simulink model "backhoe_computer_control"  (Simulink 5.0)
settings: Solver=ode5  StartTime=0.0  StopTime=inf  FixedStep=0.001  RelTol=1e-3
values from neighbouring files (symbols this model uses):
  a1 = 8.5    [startup.m]
  a2 = 48    [startup.m]
  a3 = 38+11/16    (= 38.6875)    [startup.m]
  a4 = 18.5    [startup.m]
  Butter_Order = 2    [startup.m]
  c1 = [-0.0009634 -0.4050766 2.3355377]    [startup.m]
  c2 = [ -0.00644514 2.23812750 22.79925627]    [startup.m]
  c3 = [-0.0057802 2.2376391 22.8266324]    [startup.m]
  c4 = [-0.0020828 1.5286223 20.3434998]    [startup.m]
  R1A = 10    [startup.m]
  R1B = 35.875    [startup.m]
  R2C = 36    [startup.m]
  R2D = 9+7/8    (= 9.875)    [startup.m]
  R3F = 4.5    [startup.m]
  R3G = 5.5    [startup.m]
  REF = 29.625    [startup.m]
  RFH = 9.5    [startup.m]
  RGH = 9.5    [startup.m]
  T01A = acos(RAJ/R1A)    [startup.m]
  T12C = acos((a2^2 + R2C^2 - R1C^2)/(2*a2*R2C))    [startup.m]
  T23D = 0.1317    [startup.m]
  TB12 = acos((R1B^2 + a2^2 - R2B^2)/(2*a2*R1B))    [startup.m]
  TD23 = acos((R2D^2 + a3^2 - R3D^2)/(2*a3*R2D))    [startup.m]
  TDFE = 0.0503    [startup.m]
  TG34 = 1.6966    [startup.m]
undefined symbols (not defined in the file or in its folder): channels, ended, Single
libraries: dsparch4 x18, xpclib x5, simulink x5

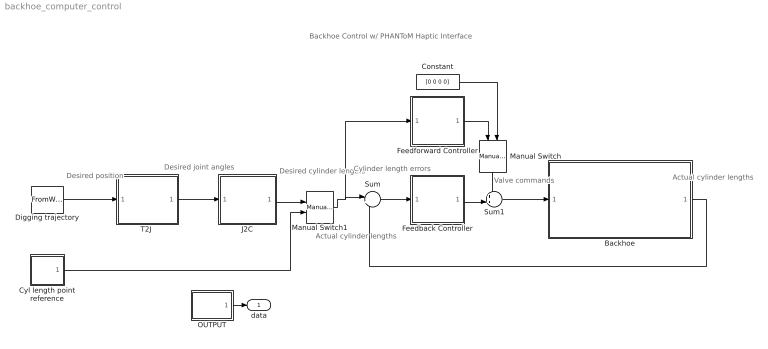
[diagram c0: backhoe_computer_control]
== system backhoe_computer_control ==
  note: Desired cylinder lengths
  note: Cylinder length errors
  note: Actual cylinder lengths
  note: Actual cylinder lengths
  note: Desired joint angles
  note: Desired position
  note: Backhoe Control w/ PHANToM Haptic Interface
  note: Valve commands
  Backhoe : Subsystem
  Constant : Constant  Value=[0 0 0 0]
  Cyl length point reference : Subsystem
  Digging trajectory : FromWorkspace  VariableName=traj  SampleTime=0  OutputAfterFinalValue=Holding final value
  Feedback Controller : Subsystem
  Feedforward Controller : Subsystem
  J2C : Subsystem
  Manual Switch : simulink/Signal Routing/Manual Switch  Orientation=down  sw=0  action=0
  Manual Switch1 : simulink/Signal Routing/Manual Switch  sw=0  action=0
  OUTPUT : Subsystem
  Sum : Sum  Inputs=|+-
  Sum1 : Sum  Inputs=++|
  "T2J " : Subsystem
  data : Outport
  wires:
  Sum/1 -> Feedback Controller/1(e)
  Backhoe/1(yc) -> Sum/2
  "T2J "/1(qdes) -> J2C/1(qdes)
  Feedback Controller/1(Us) -> Sum1/2
  Sum1/1 -> Backhoe/1(Us)
  Manual Switch/1 -> Sum1/1
  Feedforward Controller/1(UsFF) -> Manual Switch/1
  Constant/1 -> Manual Switch/2
  Digging trajectory/1 -> "T2J "/1(yp)
  J2C/1(ycdes) -> Manual Switch1/1
  Manual Switch1/1 -> Sum/1, Feedforward Controller/1(ycdes)
  Cyl length point reference/1(ycdes) -> Manual Switch1/2
  OUTPUT/1(datalog) -> data/1

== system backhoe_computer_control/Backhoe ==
  note: Valve commands
  note: Position sensor signals
  note: Cylinder lengths
  Us : Inport
  Anti-Deadband Block : Subsystem
  Backhoe Interface : Subsystem
  Position sensor conversions : Subsystem
  "Vpres -> p  conversion" : Lookup  InputValues=[2 10]  OutputValues=[0 3000]  ShowAdditionalParam=on  LookUpMeth=Interpolation-Use End Values
  yc : Outport
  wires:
  Backhoe Interface/1(Vpos) -> Position sensor conversions/1(Vc)
  Position sensor conversions/1(yc) -> yc/1, [GLOBAL_yc]
  Us/1 -> Anti-Deadband Block/1(us)
  Backhoe Interface/2(Vpres) -> "Vpres -> p  conversion"/1
  Anti-Deadband Block/1(Us) -> Backhoe Interface/1(Us)
  "Vpres -> p  conversion"/1 -> [GLOBAL_p]

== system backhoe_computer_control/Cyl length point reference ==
  Boom : Sin  Amplitude=0  Bias=31  Frequency=2*pi*0.1  SampleTime=0
  Bucket : Sin  Amplitude=0  Bias=32  Frequency=2*pi*0.1  SampleTime=0
  Mux2 : Mux
  Stick : Sin  Amplitude=0  Bias=33  Frequency=2*pi*0.1  SampleTime=0
  Swing : Sin  Amplitude=0  Frequency=2*pi*0.1  SampleTime=0
  ycdes : Outport
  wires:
  Swing/1 -> Mux2/1
  Bucket/1 -> Mux2/4
  Stick/1 -> Mux2/3
  Boom/1 -> Mux2/2
  Mux2/1 -> ycdes/1

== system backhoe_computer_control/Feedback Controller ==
  e : Inport
  Demux : Demux
  Mux : Mux
  "boom [in/s] -> [V]" : Lookup  InputValues=[-1 0 1]  OutputValues=[-0.05 0 0.6]  ShowAdditionalParam=on
  "bucket [in/s] -> [V]" : Lookup  InputValues=[-1 0 1]  OutputValues=[-0.2 0 0.2]  ShowAdditionalParam=on
  "stick [in/s] -> [V]" : Lookup  InputValues=[-1 0 1]  OutputValues=[-0.2 0 0.2]  ShowAdditionalParam=on
  "swing [rad/s] -> [V]" : Lookup  InputValues=[-1 0 1]  OutputValues=[-0.2 0 0.2]  ShowAdditionalParam=on
  Us : Outport
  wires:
  e/1 -> Demux/1
  Demux/1 -> "swing [rad/s] -> [V]"/1
  "swing [rad/s] -> [V]"/1 -> Mux/1
  Demux/2 -> "boom [in/s] -> [V]"/1
  "boom [in/s] -> [V]"/1 -> Mux/2
  Demux/3 -> "stick [in/s] -> [V]"/1
  "stick [in/s] -> [V]"/1 -> Mux/3
  Demux/4 -> "bucket [in/s] -> [V]"/1
  "bucket [in/s] -> [V]"/1 -> Mux/4
  Mux/1 -> Us/1

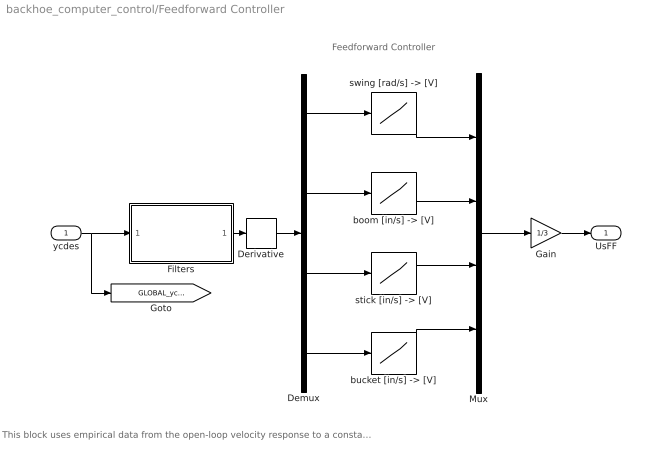
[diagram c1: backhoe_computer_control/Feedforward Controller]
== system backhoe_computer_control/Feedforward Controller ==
  note: This block uses empirical data from the open-loop velocity response to a constant voltage command to the valves. Relationships have been inverted to determine the required voltage to produce a desired velocity for each function.
  note: Feedforward Controller
  ycdes : Inport
  Demux : Demux
  Derivative : Derivative
  Filters : Subsystem
  Gain : Gain  Gain=1/3
  Mux : Mux
  "boom [in/s] -> [V]" : Lookup  InputValues=[-1.0 0 3.0]  OutputValues=[-0.25 0 0.25]  ShowAdditionalParam=on
  "bucket [in/s] -> [V]" : Lookup  InputValues=[-2.3 0 2.75]  OutputValues=[-0.25 0 0.25]  ShowAdditionalParam=on
  "stick [in/s] -> [V]" : Lookup  InputValues=[-1.6 0 1.75]  OutputValues=[-0.25 0 0.25]  ShowAdditionalParam=on
  "swing [rad/s] -> [V]" : Lookup  InputValues=[-0.6 0 0.7]  OutputValues=[-0.25 0 0.25]  ShowAdditionalParam=on
  UsFF : Outport
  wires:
  ycdes/1 -> Filters/1(unfiltered), [GLOBAL_ycdes]
  Derivative/1 -> Demux/1
  Demux/1 -> "swing [rad/s] -> [V]"/1
  "swing [rad/s] -> [V]"/1 -> Mux/1
  Demux/2 -> "boom [in/s] -> [V]"/1
  "boom [in/s] -> [V]"/1 -> Mux/2
  Demux/3 -> "stick [in/s] -> [V]"/1
  "stick [in/s] -> [V]"/1 -> Mux/3
  Demux/4 -> "bucket [in/s] -> [V]"/1
  "bucket [in/s] -> [V]"/1 -> Mux/4
  Mux/1 -> Gain/1
  Filters/1(filtered) -> Derivative/1
  Gain/1 -> UsFF/1

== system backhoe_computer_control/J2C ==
  note: Joint Space -> Cylinder Space Transformation
  note: Swing Cylinders
  qdes : Inport
  Boom cylinder : Subsystem
  Bucket cylinder : Subsystem
  Demux : Demux
  Mux : Mux
  Stick cylinder : Subsystem
  overswing  protection : Saturate  UpperLimit=pi/3  LowerLimit=-pi/2
  ycdes : Outport
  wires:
  qdes/1 -> Demux/1
  Mux/1 -> ycdes/1
  Demux/2 -> Boom cylinder/1(q2)
  Boom cylinder/1(yc3) -> Mux/2
  Demux/3 -> Stick cylinder/1(q3)
  Stick cylinder/1(yc4) -> Mux/3
  Demux/4 -> Bucket cylinder/1(q4)
  Bucket cylinder/1(yc5) -> Mux/4
  Demux/1 -> overswing  protection/1
  overswing  protection/1 -> Mux/1

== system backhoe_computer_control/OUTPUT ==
  Clock : Clock
  Mux : Mux  Inputs=5
  "Scope (xPC) " : xpclib/Misc./Scope (xPC)   scopeno=2  scopetype=Target  viewmode=Graphical redraw  grid=on  ylimits=[0,0]  autostart=on  nosamples=500  noprepostsamples=0  interleave=1  triggermode=FreeRun  triggersignal=1  triggerlevel=0.0  triggerslope=either  triggerscope=1  triggersample=0
  Scope (xPC) 1 : xpclib/Misc./Scope (xPC)   scopeno=3  scopetype=Target  viewmode=Graphical redraw  grid=on  ylimits=[0,0]  autostart=on  nosamples=500  noprepostsamples=0  interleave=1  triggermode=FreeRun  triggersignal=1  triggerlevel=0.0  triggerslope=either  triggerscope=1  triggersample=0
  Scope (xPC) 2 : xpclib/Misc./Scope (xPC)   scopeno=1  scopetype=Target  viewmode=Graphical redraw  grid=on  ylimits=[0,0]  autostart=on  nosamples=500  noprepostsamples=0  interleave=1  triggermode=FreeRun  triggersignal=1  triggerlevel=0.0  triggerslope=either  triggerscope=1  triggersample=0
  Selector : Selector  InputPortWidth=4
  datalog : Outport
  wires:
  [GLOBAL_ycdes] -> Mux/2
  Mux/1 -> datalog/1
  [GLOBAL_Us] -> Mux/3, "Scope (xPC) "/1
  [GLOBAL_yc] -> Mux/4, Selector/1
  [GLOBAL_p] -> Mux/5, Scope (xPC) 1/1
  Clock/1 -> Mux/1
  Selector/1 -> Scope (xPC) 2/1

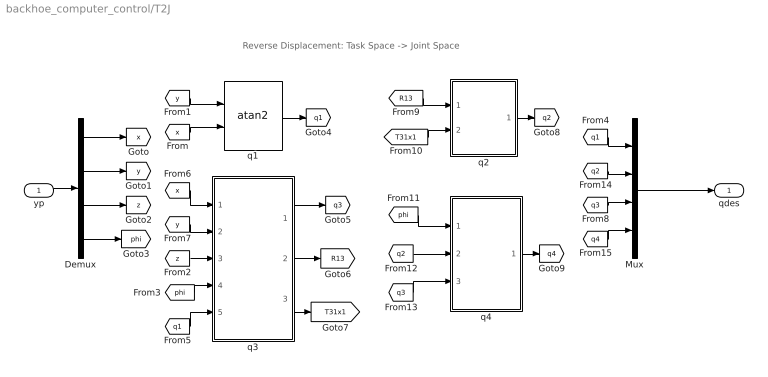
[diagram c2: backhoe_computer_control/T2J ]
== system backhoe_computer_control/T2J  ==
  note: Reverse Displacement: Task Space -> Joint Space
  yp : Inport
  Demux : Demux
  Mux : Mux
  q1 : Trigonometry  Operator=atan2
  q2 : Subsystem
  q3 : Subsystem
  q4 : Subsystem
  qdes : Outport
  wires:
  [x] -> q3/1(x)
  [y] -> q3/2(y)
  [z] -> q3/3(z)
  [phi] -> q3/4(phi)
  [q1] -> q3/5(q1)
  q3/1(q3) -> [q3]
  q3/2(R13) -> [R13]
  [y] -> q1/1
  [x] -> q1/2
  q1/1 -> [q1]
  q3/3(T31x1) -> [T31x1]
  [R13] -> q2/1(R13)
  [T31x1] -> q2/2(T31x1)
  [q3] -> q4/3(q3)
  [q2] -> q4/2(q2)
  [phi] -> q4/1(phi)
  q2/1(q2) -> [q2]
  q4/1(q4) -> [q4]
  Mux/1 -> qdes/1
  [q1] -> Mux/1
  [q3] -> Mux/3
  [q2] -> Mux/2
  [q4] -> Mux/4
  yp/1 -> Demux/1
  Demux/1 -> [x]
  Demux/2 -> [y]
  Demux/3 -> [z]
  Demux/4 -> [phi]

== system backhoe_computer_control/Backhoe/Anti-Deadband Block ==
  note: This block take a servo commmand that saturates at +-1 and converts it into valve signals. "u" in the input signal which a 4-vector. Neutral is half the voltage supplied Vc to the valves which should 6V = 1/2 * 12V. Commands to the valve must be between 25% AND 75% of Vc where 50% is neutral or the "zero command" that tell the valve to stop flow to the valve. Neutral can either be set at 6V of measure from Channel 15.
  us : Inport
  Demux : Demux
  Look-Up Table{,1..3} (4 alike) : Lookup  InputValues=[-1 -0.02 0.02 1]  OutputValues=[3 5.45 6.55 9]  ShowAdditionalParam=on  LookUpMeth=Interpolation-Use End Values  OutDataTypeMode=double
  Mux : Mux
  Us : Outport
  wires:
  Look-Up Table/1 -> Mux/1
  Look-Up Table1/1 -> Mux/2
  Demux/1 -> Look-Up Table/1
  Demux/2 -> Look-Up Table1/1
  Demux/3 -> Look-Up Table2/1
  Look-Up Table2/1 -> Mux/3
  Demux/4 -> Look-Up Table3/1
  Look-Up Table3/1 -> Mux/4
  Mux/1 -> Us/1
  us/1 -> Demux/1

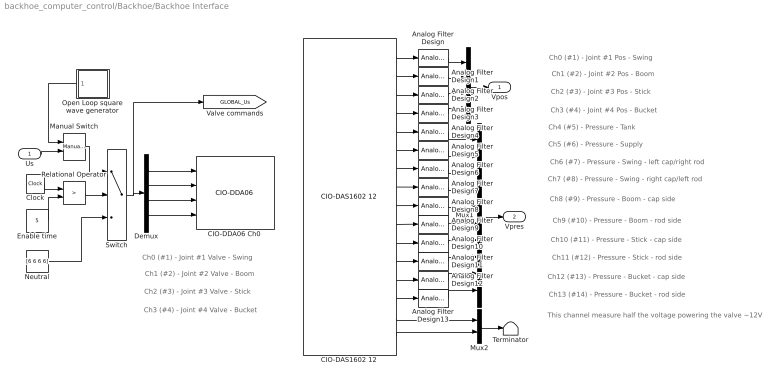
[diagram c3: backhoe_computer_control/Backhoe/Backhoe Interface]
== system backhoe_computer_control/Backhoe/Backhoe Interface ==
  note: Ch0 (#1) - Joint #1 Valve - Swing
  note: Ch1 (#2) - Joint #2 Valve - Boom
  note: Ch2 (#3) - Joint #3 Valve - Stick
  note: Ch3 (#4) - Joint #4 Valve - Bucket
  note: Ch0 (#1) - Joint #1 Pos - Swing
  note: Ch1 (#2) - Joint #2 Pos - Boom
  note: Ch2 (#3) - Joint #3 Pos - Stick
  note: Ch3 (#4) - Joint #4 Pos - Bucket
  note: Ch4 (#5) - Pressure - Tank
  note: Ch5 (#6) - Pressure - Supply
  note: Ch6 (#7) - Pressure - Swing - left cap/right rod
  note: Ch7 (#8) - Pressure - Swing - right cap/left rod
  note: Ch8 (#9) - Pressure - Boom - cap side
  note: Ch9 (#10) - Pressure - Boom - rod side
  note: Ch10 (#11) - Pressure - Stick - cap side
  note: Ch11 (#12) - Pressure - Stick - rod side
  note: Ch12 (#13) - Pressure - Bucket - cap side
  note: Ch13 (#14) - Pressure - Bucket - rod side
  note: This channel measure half the voltage powering the valve ~12V
  Us : Inport
  Analog Filter Design{,1..13} (14 alike) : dsparch4/Analog Filter Design  method=Butterworth  filttype=Lowpass  N=Butter_Order  Wlo=Butter_Rad  Whi=80  Rp=2  Rs=40
  "CIO-DAS1602 12 " : xpclib/A//D/Computer Boards/CIO-DAS1602 12   channel=16  range=0-10V  mux=Single-ended (16 channels)  sampletime=0.001  baseaddress=0x340
  "CIO-DDA06 Ch0 " : xpclib/D//A/Computer Boards/CIO-DDA06   channel=[1 2 3 4]  range=[10 10 10 10]  reset=[1 1 1 1]  initValue=[6 6 6 6]  sampletime=0.001  baseaddress=0x300
  Clock : Clock
  Demux : Demux
  Enable time : Constant  Value=5
  Manual Switch : simulink/Signal Routing/Manual Switch  sw=0  action=0
  Mux : Mux
  Mux1 : Mux  Inputs=10
  Mux2 : Mux  Inputs=2
  Neutral : Constant  Value=[6 6 6 6]  ShowAdditionalParam=on
  Open Loop square wave generator : Subsystem  Orientation=left
  Relational Operator : RelationalOperator  Operator=>  ShowAdditionalParam=on
  Switch : Switch  Threshold=0.5  ShowAdditionalParam=on
  Terminator : Terminator
  Vpos : Outport
  Vpres : Outport  Port=2
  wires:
  Demux/2 -> "CIO-DDA06 Ch0 "/2
  Demux/3 -> "CIO-DDA06 Ch0 "/3
  Demux/4 -> "CIO-DDA06 Ch0 "/4
  Mux/1 -> Vpos/1
  "CIO-DAS1602 12 "/1 -> Analog Filter Design/1
  Analog Filter Design/1 -> Mux/1
  "CIO-DAS1602 12 "/2 -> Analog Filter Design1/1
  "CIO-DAS1602 12 "/3 -> Analog Filter Design2/1
  "CIO-DAS1602 12 "/4 -> Analog Filter Design3/1
  Analog Filter Design1/1 -> Mux/2
  Analog Filter Design2/1 -> Mux/3
  Analog Filter Design3/1 -> Mux/4
  "CIO-DAS1602 12 "/5 -> Analog Filter Design4/1
  "CIO-DAS1602 12 "/6 -> Analog Filter Design5/1
  "CIO-DAS1602 12 "/7 -> Analog Filter Design6/1
  "CIO-DAS1602 12 "/8 -> Analog Filter Design7/1
  "CIO-DAS1602 12 "/9 -> Analog Filter Design8/1
  "CIO-DAS1602 12 "/10 -> Analog Filter Design9/1
  "CIO-DAS1602 12 "/11 -> Analog Filter Design10/1
  "CIO-DAS1602 12 "/12 -> Analog Filter Design11/1
  "CIO-DAS1602 12 "/13 -> Analog Filter Design12/1
  "CIO-DAS1602 12 "/14 -> Analog Filter Design13/1
  "CIO-DAS1602 12 "/15 -> Mux2/1
  Analog Filter Design4/1 -> Mux1/1
  Analog Filter Design5/1 -> Mux1/2
  Analog Filter Design6/1 -> Mux1/3
  Analog Filter Design7/1 -> Mux1/4
  Analog Filter Design8/1 -> Mux1/5
  Analog Filter Design9/1 -> Mux1/6
  Analog Filter Design10/1 -> Mux1/7
  Analog Filter Design11/1 -> Mux1/8
  Analog Filter Design12/1 -> Mux1/9
  Analog Filter Design13/1 -> Mux1/10
  Mux1/1 -> Vpres/1
  Mux2/1 -> Terminator/1
  "CIO-DAS1602 12 "/16 -> Mux2/2
  Switch/1 -> Demux/1, [GLOBAL_Us]
  Clock/1 -> Relational Operator/1
  Enable time/1 -> Relational Operator/2
  Relational Operator/1 -> Switch/2
  Neutral/1 -> Switch/3
  Demux/1 -> "CIO-DDA06 Ch0 "/1
  Manual Switch/1 -> Switch/1
  Us/1 -> Manual Switch/2
  Open Loop square wave generator/1(UsOL) -> Manual Switch/1

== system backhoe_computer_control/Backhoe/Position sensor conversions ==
  note: Sensor Conversions
  Vc : Inport
  Boom sensor : Subsystem
  Bucket sensor : Subsystem
  Demux : Demux
  Mux : Mux
  Stick sensor : Subsystem
  Swing pot : Subsystem
  yc : Outport
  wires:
  Vc/1 -> Demux/1
  Demux/1 -> Swing pot/1(Vc1)
  Demux/2 -> Boom sensor/1(Vc2)
  Swing pot/1(q1) -> Mux/1
  Boom sensor/1(yc3) -> Mux/2
  Demux/3 -> Stick sensor/1(Vc3)
  Stick sensor/1(yc4) -> Mux/3
  Mux/1 -> yc/1
  Demux/4 -> Bucket sensor/1(Vc4)
  Bucket sensor/1(yc5) -> Mux/4

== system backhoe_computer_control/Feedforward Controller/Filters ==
  unfiltered : Inport
  Analog Filter Design{,1..3} (4 alike) : dsparch4/Analog Filter Design  method=Butterworth  filttype=Lowpass  N=2  Wlo=2*pi*5  Whi=80  Rp=2  Rs=40
  Demux : Demux
  Mux : Mux
  filtered : Outport
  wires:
  unfiltered/1 -> Demux/1
  Demux/1 -> Analog Filter Design/1
  Analog Filter Design/1 -> Mux/1
  Demux/2 -> Analog Filter Design1/1
  Analog Filter Design1/1 -> Mux/2
  Demux/3 -> Analog Filter Design2/1
  Analog Filter Design2/1 -> Mux/3
  Demux/4 -> Analog Filter Design3/1
  Analog Filter Design3/1 -> Mux/4
  Mux/1 -> filtered/1

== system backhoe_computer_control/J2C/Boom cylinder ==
  q2 : Inport
  Constant : Constant  Value=pi
  Constant1 : Constant  Value=T01A
  Constant2 : Constant  Value=TB12
  CosineLawB : Subsystem
  Sum : Sum  Inputs=+---
  yc3 : Outport
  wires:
  Constant/1 -> Sum/1
  Constant1/1 -> Sum/2
  Sum/1 -> CosineLawB/1(TA1B)
  CosineLawB/1(yc3) -> yc3/1
  q2/1 -> Sum/3
  Constant2/1 -> Sum/4

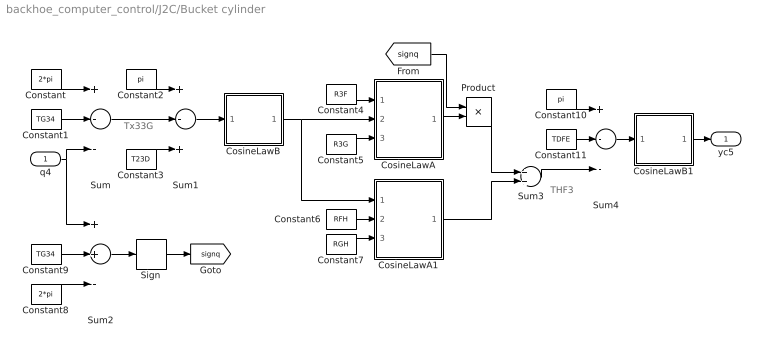
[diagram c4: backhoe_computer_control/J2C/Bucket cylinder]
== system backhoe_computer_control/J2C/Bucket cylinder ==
  note: Tx33G
  note: THF3
  q4 : Inport
  Constant : Constant  Value=2*pi
  Constant1 : Constant  Value=TG34
  Constant10 : Constant  Value=pi
  Constant11 : Constant  Value=TDFE
  Constant2 : Constant  Value=pi
  Constant3 : Constant  Value=T23D
  Constant4 : Constant  Value=R3F
  Constant5 : Constant  Value=R3G
  Constant6 : Constant  Value=RFH
  Constant7 : Constant  Value=RGH
  Constant8 : Constant  Value=2*pi
  Constant9 : Constant  Value=TG34
  CosineLawA : Subsystem
  CosineLawA1 : Subsystem
  CosineLawB : Subsystem
  CosineLawB1 : Subsystem
  Product : Product
  Sign : Signum
  Sum : Sum  Inputs=+--
  Sum1 : Sum  Inputs=+-+
  Sum2 : Sum  Inputs=++-
  Sum3 : Sum
  Sum4 : Sum  Inputs=+--
  yc5 : Outport
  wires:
  Constant/1 -> Sum/1
  Constant1/1 -> Sum/2
  Sum/1 -> Sum1/2
  Constant2/1 -> Sum1/1
  Constant3/1 -> Sum1/3
  Sum1/1 -> CosineLawB/1(TG3F)
  CosineLawB/1(rFG) -> CosineLawA/2(r2), CosineLawA1/1(r1)
  Constant4/1 -> CosineLawA/1(r1)
  Constant5/1 -> CosineLawA/3(r3)
  Constant6/1 -> CosineLawA1/2(r2)
  Constant7/1 -> CosineLawA1/3(r3)
  Constant9/1 -> Sum2/2
  Constant8/1 -> Sum2/3
  Sum2/1 -> Sign/1
  [signq] -> Product/1
  CosineLawA/1(T3FG) -> Product/2
  Sign/1 -> [signq]
  Product/1 -> Sum3/1
  CosineLawA1/1(THFG) -> Sum3/2
  Constant10/1 -> Sum4/1
  Sum3/1 -> Sum4/3
  Constant11/1 -> Sum4/2
  Sum4/1 -> CosineLawB1/1(TEFH)
  CosineLawB1/1(yc5) -> yc5/1
  q4/1 -> Sum/3, Sum2/1

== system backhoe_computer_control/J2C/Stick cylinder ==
  q3 : Inport
  Constant : Constant  Value=pi
  Constant1 : Constant  Value=TD23
  Constant2 : Constant  Value=T12C
  CosineLawB : Subsystem
  Sum : Sum  Inputs=+---
  yc4 : Outport
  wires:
  Constant/1 -> Sum/1
  Constant1/1 -> Sum/2
  Sum/1 -> CosineLawB/1(TC2D)
  CosineLawB/1(yc4) -> yc4/1
  q3/1 -> Sum/3
  Constant2/1 -> Sum/4

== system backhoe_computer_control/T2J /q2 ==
  note: T213
  R13 : Inport
  T31x1 : Inport  Port=2
  CosineLawA : Subsystem
  Sum : Sum  Inputs=|++
  a2 : Constant  Value=a2
  a3 : Constant  Value=a3
  q2 : Outport
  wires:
  a2/1 -> CosineLawA/1(r1)
  a3/1 -> CosineLawA/3(r3)
  CosineLawA/1(theta) -> Sum/1
  Sum/1 -> q2/1
  R13/1 -> CosineLawA/2(r2)
  T31x1/1 -> Sum/2

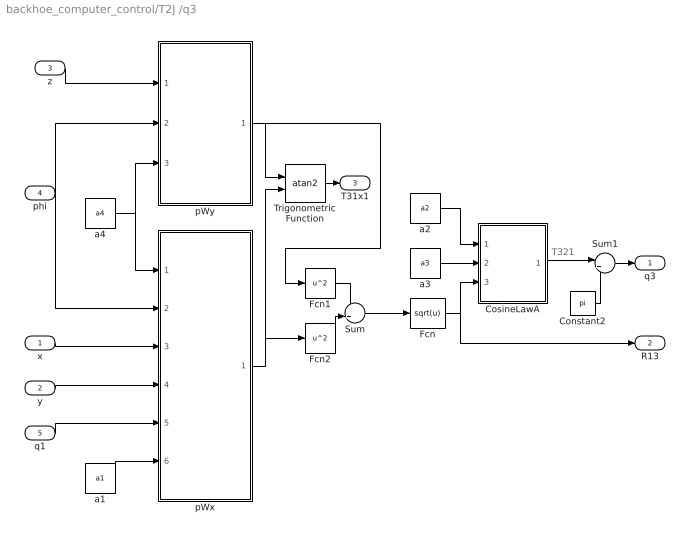
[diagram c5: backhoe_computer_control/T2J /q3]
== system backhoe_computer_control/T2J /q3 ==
  note: T321
  x : Inport
  y : Inport  Port=2
  z : Inport  Port=3
  phi : Inport  Port=4
  q1 : Inport  Port=5
  Constant2 : Constant  Value=pi
  CosineLawA : Subsystem
  Fcn : Fcn  Expr=sqrt(u)
  Fcn1 : Fcn  Expr=u^2
  Fcn2 : Fcn  Expr=u^2
  Sum : Sum
  Sum1 : Sum  Inputs=|++
  Trigonometric Function : Trigonometry  Operator=atan2
  a1 : Constant  Value=a1
  a2 : Constant  Value=a2
  a3 : Constant  Value=a3
  a4 : Constant  Value=a4
  pWx : Subsystem
  pWy : Subsystem
  q3 : Outport
  R13 : Outport  Port=2
  T31x1 : Outport  Port=3
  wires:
  a1/1 -> pWx/6(a1)
  q1/1 -> pWx/5(q1)
  y/1 -> pWx/4(y)
  x/1 -> pWx/3(x)
  a4/1 -> pWx/1(a4), pWy/3(a4)
  z/1 -> pWy/1(z)
  phi/1 -> pWx/2(phi), pWy/2(phi)
  pWy/1(pWy) -> Fcn1/1, Trigonometric Function/1
  Trigonometric Function/1 -> T31x1/1
  Fcn1/1 -> Sum/1
  Fcn2/1 -> Sum/2
  Sum/1 -> Fcn/1
  pWx/1(pWx) -> Fcn2/1, Trigonometric Function/2
  a3/1 -> CosineLawA/2(r2)
  a2/1 -> CosineLawA/1(r1)
  Fcn/1 -> CosineLawA/3(r3), R13/1
  Sum1/1 -> q3/1
  Constant2/1 -> Sum1/2
  CosineLawA/1(theta) -> Sum1/1

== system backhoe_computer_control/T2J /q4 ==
  phi : Inport
  q2 : Inport  Port=2
  q3 : Inport  Port=3
  Constant : Constant  Value=3*pi
  Sum : Sum  Inputs=+--+
  q4 : Outport
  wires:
  phi/1 -> Sum/1
  q2/1 -> Sum/2
  Sum/1 -> q4/1
  q3/1 -> Sum/3
  Constant/1 -> Sum/4

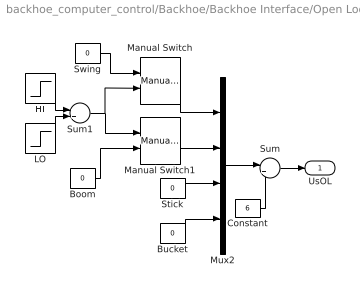
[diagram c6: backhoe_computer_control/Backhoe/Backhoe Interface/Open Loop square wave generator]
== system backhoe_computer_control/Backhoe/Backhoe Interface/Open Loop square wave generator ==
  Boom : Constant  Value=0
  Bucket : Constant  Value=0
  Constant : Constant  Value=6
  HI : Step  Time=8  After=3  SampleTime=0
  LO : Step  Time=9  After=-3  SampleTime=0
  Manual Switch : simulink/Signal Routing/Manual Switch  sw=0  action=0
  Manual Switch1 : simulink/Signal Routing/Manual Switch  sw=0  action=0
  Mux2 : Mux
  Stick : Constant  Value=0
  Sum : Sum  Inputs=|++
  Sum1 : Sum
  Swing : Constant  Value=0
  UsOL : Outport
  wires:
  Manual Switch/1 -> Mux2/1
  Bucket/1 -> Mux2/4
  Stick/1 -> Mux2/3
  Manual Switch1/1 -> Mux2/2
  Mux2/1 -> Sum/1
  Sum/1 -> UsOL/1
  Constant/1 -> Sum/2
  HI/1 -> Sum1/1
  LO/1 -> Sum1/2
  Sum1/1 -> Manual Switch/2, Manual Switch1/1
  Swing/1 -> Manual Switch/1
  Boom/1 -> Manual Switch1/2

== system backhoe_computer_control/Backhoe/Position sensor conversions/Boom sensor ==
  Vc2 : Inport
  Fcn : Fcn  Expr=u^2
  Product : Product
  Product1 : Product
  Sum : Sum  Inputs=+++
  c10 : Constant  Value=c2(3)
  c11 : Constant  Value=c2(2)
  c12 : Constant  Value=c2(1)
  yc3 : Outport
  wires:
  Vc2/1 -> Fcn/1, Product1/2
  Product1/1 -> Sum/2
  c10/1 -> Sum/3
  c12/1 -> Product/1
  Fcn/1 -> Product/2
  Product/1 -> Sum/1
  c11/1 -> Product1/1
  Sum/1 -> yc3/1

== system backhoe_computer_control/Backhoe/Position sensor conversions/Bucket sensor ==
  Vc4 : Inport
  Fcn : Fcn  Expr=u^2
  Product : Product
  Product1 : Product
  Sum : Sum  Inputs=+++
  c10 : Constant  Value=c4(3)
  c11 : Constant  Value=c4(2)
  c12 : Constant  Value=c4(1)
  yc5 : Outport
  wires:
  Vc4/1 -> Fcn/1, Product1/2
  Product1/1 -> Sum/2
  c10/1 -> Sum/3
  c12/1 -> Product/1
  Fcn/1 -> Product/2
  Product/1 -> Sum/1
  c11/1 -> Product1/1
  Sum/1 -> yc5/1

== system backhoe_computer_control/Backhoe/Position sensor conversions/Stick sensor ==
  Vc3 : Inport
  Fcn : Fcn  Expr=u^2
  Product : Product
  Product1 : Product
  Sum : Sum  Inputs=+++
  c10 : Constant  Value=c3(3)
  c11 : Constant  Value=c3(2)
  c12 : Constant  Value=c3(1)
  yc4 : Outport
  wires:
  Vc3/1 -> Fcn/1, Product1/2
  Product1/1 -> Sum/2
  c10/1 -> Sum/3
  c12/1 -> Product/1
  Fcn/1 -> Product/2
  Product/1 -> Sum/1
  c11/1 -> Product1/1
  Sum/1 -> yc4/1

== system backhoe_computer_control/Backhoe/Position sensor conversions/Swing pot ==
  Vc1 : Inport
  Fcn : Fcn  Expr=u^2
  Product : Product
  Product1 : Product
  Sum : Sum  Inputs=+++
  c10 : Constant  Value=c1(3)
  c11 : Constant  Value=c1(2)
  c12 : Constant  Value=c1(1)
  q1 : Outport
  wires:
  Vc1/1 -> Fcn/1, Product1/2
  Product1/1 -> Sum/2
  c10/1 -> Sum/3
  c12/1 -> Product/1
  Fcn/1 -> Product/2
  Product/1 -> Sum/1
  c11/1 -> Product1/1
  Sum/1 -> q1/1

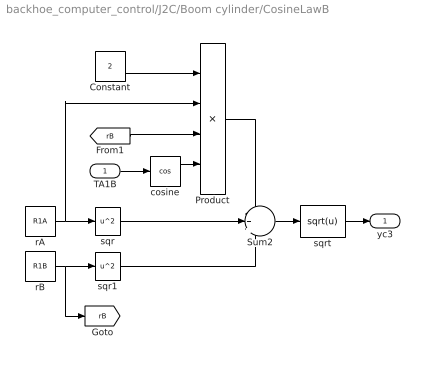
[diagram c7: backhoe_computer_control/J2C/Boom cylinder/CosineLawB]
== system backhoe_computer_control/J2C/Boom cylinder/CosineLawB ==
  TA1B : Inport
  Constant : Constant  Value=2
  Product : Product  Inputs=4
  Sum2 : Sum  Inputs=-++
  cosine : Trigonometry  Operator=cos
  rA : Constant  Value=R1A
  rB : Constant  Value=R1B
  sqr : Fcn  Expr=u^2
  sqr1 : Fcn  Expr=u^2
  sqrt : Fcn  Expr=sqrt(u)
  yc3 : Outport
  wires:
  rA/1 -> sqr/1, Product/2
  sqr1/1 -> Sum2/3
  Constant/1 -> Product/1
  [rB] -> Product/3
  sqr/1 -> Sum2/2
  Product/1 -> Sum2/1
  cosine/1 -> Product/4
  Sum2/1 -> sqrt/1
  TA1B/1 -> cosine/1
  sqrt/1 -> yc3/1
  rB/1 -> sqr1/1, [rB]

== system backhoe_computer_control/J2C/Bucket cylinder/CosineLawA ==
  r1 : Inport
  r2 : Inport  Port=2
  r3 : Inport  Port=3
  Fcn1 : Fcn  Expr=u^2
  Fcn2 : Fcn  Expr=u^2
  Fcn3 : Fcn  Expr=u^2
  Gain : Gain  Gain=2
  Product : Product
  Product1 : Product  Inputs=*/
  Sum : Sum  Inputs=++-
  Trigonometric Function : Trigonometry  Operator=acos
  T3FG : Outport
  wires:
  r3/1 -> Fcn3/1
  Fcn1/1 -> Sum/1
  Fcn2/1 -> Sum/2
  Fcn3/1 -> Sum/3
  r2/1 -> Fcn2/1, Product/1
  r1/1 -> Fcn1/1, Product/2
  Product/1 -> Gain/1
  Sum/1 -> Product1/1
  Gain/1 -> Product1/2
  Product1/1 -> Trigonometric Function/1
  Trigonometric Function/1 -> T3FG/1

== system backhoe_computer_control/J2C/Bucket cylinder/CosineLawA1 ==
  r1 : Inport
  r2 : Inport  Port=2
  r3 : Inport  Port=3
  Fcn1 : Fcn  Expr=u^2
  Fcn2 : Fcn  Expr=u^2
  Fcn3 : Fcn  Expr=u^2
  Gain : Gain  Gain=2
  Product : Product
  Product1 : Product  Inputs=*/
  Sum : Sum  Inputs=++-
  Trigonometric Function : Trigonometry  Operator=acos
  THFG : Outport
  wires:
  r3/1 -> Fcn3/1
  Fcn1/1 -> Sum/1
  Fcn2/1 -> Sum/2
  Fcn3/1 -> Sum/3
  r2/1 -> Fcn2/1, Product/1
  r1/1 -> Fcn1/1, Product/2
  Product/1 -> Gain/1
  Sum/1 -> Product1/1
  Gain/1 -> Product1/2
  Product1/1 -> Trigonometric Function/1
  Trigonometric Function/1 -> THFG/1

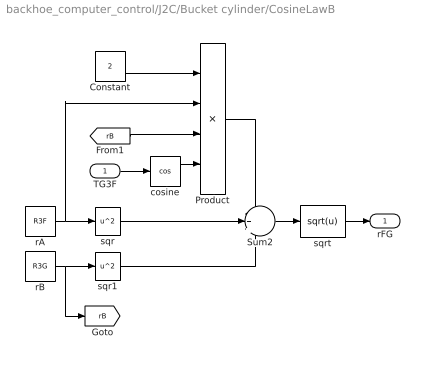
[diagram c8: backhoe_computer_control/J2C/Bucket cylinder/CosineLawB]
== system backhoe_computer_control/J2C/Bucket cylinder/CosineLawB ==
  TG3F : Inport
  Constant : Constant  Value=2
  Product : Product  Inputs=4
  Sum2 : Sum  Inputs=-++
  cosine : Trigonometry  Operator=cos
  rA : Constant  Value=R3F
  rB : Constant  Value=R3G
  sqr : Fcn  Expr=u^2
  sqr1 : Fcn  Expr=u^2
  sqrt : Fcn  Expr=sqrt(u)
  rFG : Outport
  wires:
  rA/1 -> sqr/1, Product/2
  sqr1/1 -> Sum2/3
  Constant/1 -> Product/1
  [rB] -> Product/3
  sqr/1 -> Sum2/2
  Product/1 -> Sum2/1
  cosine/1 -> Product/4
  Sum2/1 -> sqrt/1
  TG3F/1 -> cosine/1
  sqrt/1 -> rFG/1
  rB/1 -> sqr1/1, [rB]

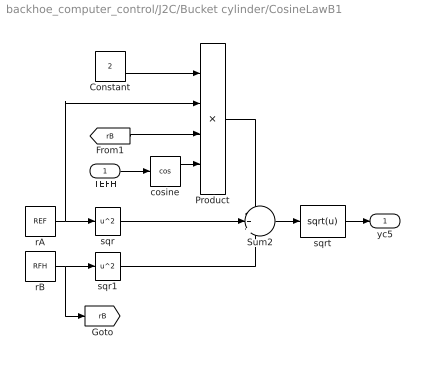
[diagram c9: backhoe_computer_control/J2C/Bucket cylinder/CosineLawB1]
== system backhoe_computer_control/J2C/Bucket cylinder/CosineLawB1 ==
  TEFH : Inport
  Constant : Constant  Value=2
  Product : Product  Inputs=4
  Sum2 : Sum  Inputs=-++
  cosine : Trigonometry  Operator=cos
  rA : Constant  Value=REF
  rB : Constant  Value=RFH
  sqr : Fcn  Expr=u^2
  sqr1 : Fcn  Expr=u^2
  sqrt : Fcn  Expr=sqrt(u)
  yc5 : Outport
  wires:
  rA/1 -> sqr/1, Product/2
  sqr1/1 -> Sum2/3
  Constant/1 -> Product/1
  [rB] -> Product/3
  sqr/1 -> Sum2/2
  Product/1 -> Sum2/1
  cosine/1 -> Product/4
  Sum2/1 -> sqrt/1
  TEFH/1 -> cosine/1
  sqrt/1 -> yc5/1
  rB/1 -> sqr1/1, [rB]

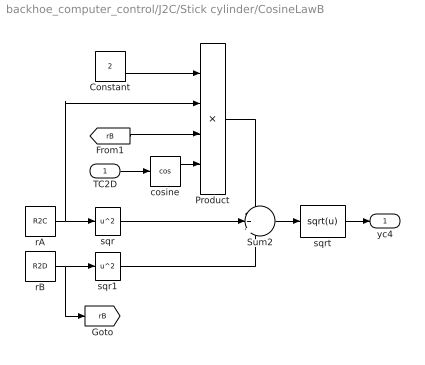
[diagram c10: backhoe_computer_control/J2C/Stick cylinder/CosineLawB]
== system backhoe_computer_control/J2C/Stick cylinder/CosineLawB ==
  TC2D : Inport
  Constant : Constant  Value=2
  Product : Product  Inputs=4
  Sum2 : Sum  Inputs=-++
  cosine : Trigonometry  Operator=cos
  rA : Constant  Value=R2C
  rB : Constant  Value=R2D
  sqr : Fcn  Expr=u^2
  sqr1 : Fcn  Expr=u^2
  sqrt : Fcn  Expr=sqrt(u)
  yc4 : Outport
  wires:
  rA/1 -> sqr/1, Product/2
  sqr1/1 -> Sum2/3
  Constant/1 -> Product/1
  [rB] -> Product/3
  sqr/1 -> Sum2/2
  Product/1 -> Sum2/1
  cosine/1 -> Product/4
  Sum2/1 -> sqrt/1
  TC2D/1 -> cosine/1
  sqrt/1 -> yc4/1
  rB/1 -> sqr1/1, [rB]

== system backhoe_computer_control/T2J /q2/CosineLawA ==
  r1 : Inport
  r2 : Inport  Port=2
  r3 : Inport  Port=3
  Fcn1 : Fcn  Expr=u^2
  Fcn2 : Fcn  Expr=u^2
  Fcn3 : Fcn  Expr=u^2
  Gain : Gain  Gain=2
  Product : Product
  Product1 : Product  Inputs=*/
  Sum : Sum  Inputs=++-
  Trigonometric Function : Trigonometry  Operator=acos
  theta : Outport
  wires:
  r3/1 -> Fcn3/1
  Fcn1/1 -> Sum/1
  Fcn2/1 -> Sum/2
  Fcn3/1 -> Sum/3
  r2/1 -> Fcn2/1, Product/1
  r1/1 -> Fcn1/1, Product/2
  Product/1 -> Gain/1
  Sum/1 -> Product1/1
  Gain/1 -> Product1/2
  Product1/1 -> Trigonometric Function/1
  Trigonometric Function/1 -> theta/1

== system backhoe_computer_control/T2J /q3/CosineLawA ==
  r1 : Inport
  r2 : Inport  Port=2
  r3 : Inport  Port=3
  Fcn1 : Fcn  Expr=u^2
  Fcn2 : Fcn  Expr=u^2
  Fcn3 : Fcn  Expr=u^2
  Gain : Gain  Gain=2
  Product : Product
  Product1 : Product  Inputs=*/
  Sum : Sum  Inputs=++-
  Trigonometric Function : Trigonometry  Operator=acos
  theta : Outport
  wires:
  r3/1 -> Fcn3/1
  Fcn1/1 -> Sum/1
  Fcn2/1 -> Sum/2
  Fcn3/1 -> Sum/3
  r2/1 -> Fcn2/1, Product/1
  r1/1 -> Fcn1/1, Product/2
  Product/1 -> Gain/1
  Sum/1 -> Product1/1
  Gain/1 -> Product1/2
  Product1/1 -> Trigonometric Function/1
  Trigonometric Function/1 -> theta/1

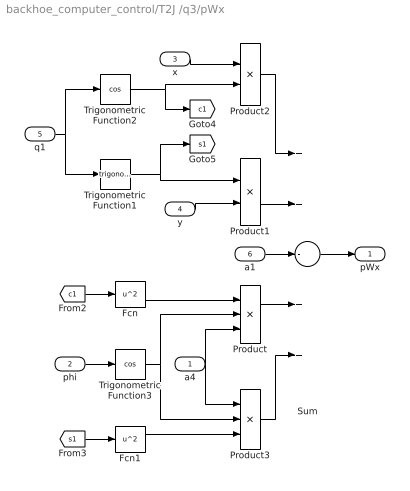
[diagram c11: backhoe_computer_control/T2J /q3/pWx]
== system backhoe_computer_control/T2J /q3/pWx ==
  a4 : Inport
  phi : Inport  Port=2
  x : Inport  Port=3
  y : Inport  Port=4
  q1 : Inport  Port=5
  a1 : Inport  Port=6
  Fcn : Fcn  Expr=u^2
  Fcn1 : Fcn  Expr=u^2
  Product : Product  Inputs=3
  Product1 : Product
  Product2 : Product
  Product3 : Product  Inputs=3
  Sum : Sum  Inputs=++-++
  Trigonometric Function1 : Trigonometry
  Trigonometric Function2 : Trigonometry  Operator=cos
  Trigonometric Function3 : Trigonometry  Operator=cos
  pWx : Outport
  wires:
  Product2/1 -> Sum/1
  Product1/1 -> Sum/2
  x/1 -> Product2/1
  Sum/1 -> pWx/1
  a1/1 -> Sum/3
  q1/1 -> Trigonometric Function2/1, Trigonometric Function1/1
  y/1 -> Product1/2
  Trigonometric Function1/1 -> Product1/1, [s1]
  Trigonometric Function2/1 -> Product2/2, [c1]
  Product/1 -> Sum/4
  Product3/1 -> Sum/5
  [c1] -> Fcn/1
  Fcn/1 -> Product/1
  a4/1 -> Product/3, Product3/1
  Trigonometric Function3/1 -> Product/2, Product3/2
  Fcn1/1 -> Product3/3
  [s1] -> Fcn1/1
  phi/1 -> Trigonometric Function3/1

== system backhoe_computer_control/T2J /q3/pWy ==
  z : Inport
  phi : Inport  Port=2
  a4 : Inport  Port=3
  Product : Product
  Sum : Sum  Inputs=|++
  Trigonometric Function : Trigonometry
  pWy : Outport
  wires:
  Trigonometric Function/1 -> Product/2
  a4/1 -> Product/1
  Product/1 -> Sum/1
  Sum/1 -> pWy/1
  phi/1 -> Trigonometric Function/1
  z/1 -> Sum/2
